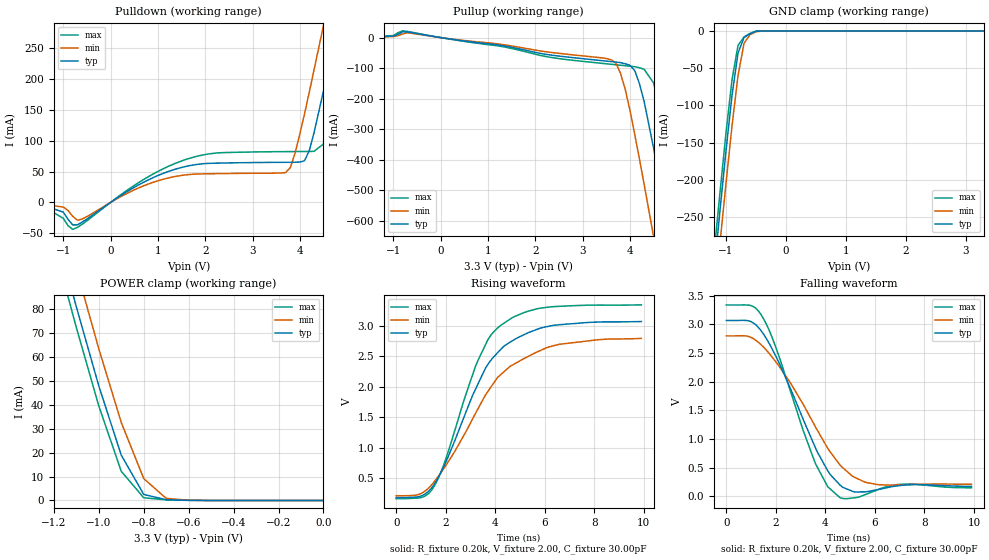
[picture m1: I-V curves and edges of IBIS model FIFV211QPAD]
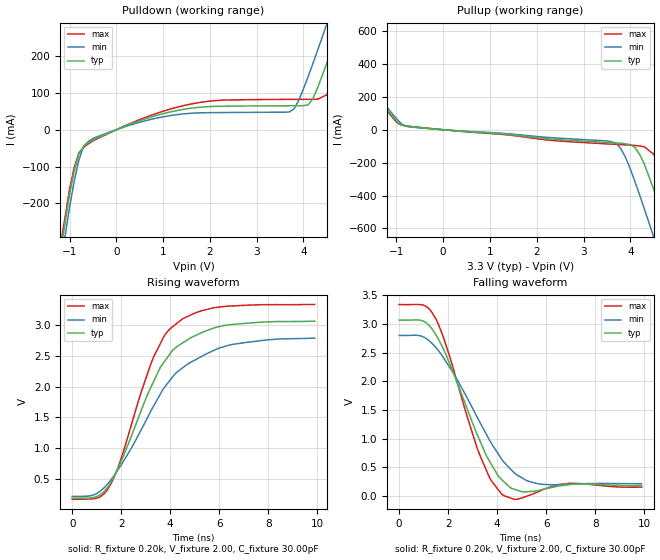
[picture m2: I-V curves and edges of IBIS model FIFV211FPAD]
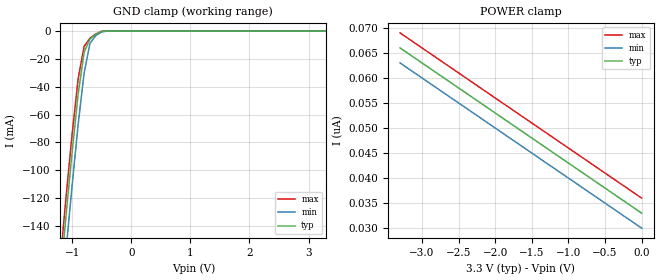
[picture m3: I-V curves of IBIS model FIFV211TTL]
| IBIS file i72v801.ibs created by s2ibis2 version 1.1
| North Carolina State University Electronics Research Laboratory  1995
[IBIS ver]   2.1
[File name]   i72v801.ibs
[File Rev]   1.0
[Date]   06/08/98
[Source]   Integrated Device Technology, Inc.
[Notes]   1. Temperatures: typ=25C, min=70C, max=0C 2. Cemos8_3.3v
   process. 3. Ramp rates based on 50 ohm load.
[Copyright]   Copyright 1998, Integrated Device Technology, Inc.
|   Component idt72V801
[Component]   idt72V801
[Manufacturer]   Integrated Device Technology
[Package]
| variable   typ   min   max
R_pkg   0.75   0.60   0.90
L_pkg   8.10nH   8.30nH   9.90nH
C_pkg   0.53pF   0.46pF   0.60pF
[Pin]  signal_name   model_name   R_pin   L_pin   C_pin
1   QA1   FIFV211QPAD
2   QA2   FIFV211QPAD
3   QA3   FIFV211QPAD
4   QA4   FIFV211QPAD
5   QA5   FIFV211QPAD
6   QA6   FIFV211QPAD
7   QA7   FIFV211QPAD
8   QA8   FIFV211QPAD
9   VCC   POWER
10   WENA2   FIFV211TTL
11   WCLKA   FIFV211TTL
12   WENAL1   FIFV211TTL
13   RSAL   FIFV211TTL
14   DA8   FIFV211TTL
15   DA7   FIFV211TTL
16   DA6   FIFV211TTL
17   DA5   FIFV211TTL
18   DA4   FIFV211TTL
19   DA3   FIFV211TTL
20   DA2   FIFV211TTL
21   DA1   FIFV211TTL
22   DA0   FIFV211TTL
23   PAFAL   FIFV211FPAD
24   PAEAL   FIFV211FPAD
25   WENB2   FIFV211TTL
26   WCLKB   FIFV211TTL
27   WENBL1   FIFV211TTL
28   RSBL   FIFV211TTL
29   DB8   FIFV211TTL
30   DB7   FIFV211TTL
31   DB6   FIFV211TTL
32   DB5   FIFV211TTL
33   DB4   FIFV211TTL
34   DB3   FIFV211TTL
35   DB2   FIFV211TTL
36   DB1   FIFV211TTL
37   DB0   FIFV211TTL
38   PAFBL   FIFV211FPAD
39   PAEBL   FIFV211FPAD
40   VCC   POWER
41   GND   GND
42   RENBL1   FIFV211TTL
43   RCLKB   FIFV211TTL
44   RENBL2   FIFV211TTL
45   OEBL   FIFV211TTL
46   EFBL   FIFV211FPAD
47   FFBL   FIFV211FPAD
48   QB0   FIFV211QPAD
49   QB1   FIFV211QPAD
50   QB2   FIFV211QPAD
51   QB3   FIFV211QPAD
52   QB4   FIFV211QPAD
53   QB5   FIFV211QPAD
54   QB6   FIFV211QPAD
55   QB7   FIFV211QPAD
56   QB8   FIFV211QPAD
57   GND   GND
58   RENAL1   FIFV211TTL
59   RCLKA   FIFV211TTL
60   RENAL2   FIFV211TTL
61   OEAL   FIFV211TTL
62   EFAL   FIFV211FPAD
63   FFAL   FIFV211FPAD
64   QA0   FIFV211QPAD
| Models and submodels in the file (3): FIFV211QPAD (3-state), FIFV211FPAD (Output), FIFV211TTL (Input)
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| FIN  FIN   dummy_model
| QIN  QIN   dummy_model
| QOEL QOEL   dummy_model
|   Model FIFV211QPAD
[Model]   FIFV211QPAD
Model_type   3-state
Polarity   Non-Inverting
Enable   Active-Low
Vmeas =  1.500V
C_comp   3.00pF   NA   NA
[Temperature Range]   25.00   70.00   0.000
[Voltage Range]   3.30V   3.00V   3.60V
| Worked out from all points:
|   slope of the pulldown table from 0 to 0.495 V, typ, clamps not added: 20.4 ohm
|   slope of the pullup table from 0 to 0.495 V, typ, clamps not added: 44.7 ohm
|   GND clamp passes 1 mA (typ) near -0.52 V on its own axis
|   POWER clamp passes 1 mA (typ) near -0.73 V on its own axis
|   rising waveform, R_fixture 0.20k, V_fixture 2.00, C_fixture 30.00pF: 20-80 % time 1.95ns typ, 2.41ns min, 1.64ns max; typ from 0.181 V to 3.07 V
|   falling waveform, R_fixture 0.20k, V_fixture 2.00, C_fixture 30.00pF: 20-80 % time 1.76ns typ, 2.17ns min, 1.5ns max; typ from 3.07 V to 0.177 V
[Pulldown]
| voltage   I(typ)   I(min)   I(max)
-3.3V     -1mA       -1mA       0A
-1.5V     -2.7mA     -2.1mA     -3.3mA
-800mV    -36.55mA   -22.69mA   -43.77mA
1.5V      56.64mA    43.75mA    67.16mA
3.7V      65mA       48.37mA    82.35mA
3.9V      65.11mA    80.12mA    82.43mA
4.1V      67.6mA     144mA      82.48mA
4.5V      181mA      287mA      94.75mA
4.7V      253mA      361mA      155mA
4.9V      326mA      435mA      225mA
5.1V      400mA      510mA      298mA
6.6V      966mA      1.076A     862mA
[Pullup]
| voltage   I(typ)   I(min)   I(max)
-3.3V     300uA      300uA      300uA
-800mV    19.13mA    12.44mA    22.38mA
3.6V      -78.68mA   -72.88mA   -87.52mA
3.7V      -80.24mA   -82.94mA   -89.09mA
3.9V      -85.87mA   -170mA     -92.22mA
4.1V      -108mA     -317mA     -95.4mA
4.3V      -210mA     -482mA     -104mA
4.5V      -363mA     -653mA     -149mA
4.7V      -531mA     -826mA     -270mA
4.9V      -703mA     -1A        -430mA
5.1V      -878mA     -1.176A    -601mA
6.6V      -2.207A    -2.508A    -1.926A
[GND_clamp]
| voltage   I(typ)   I(min)   I(max)
-3.3V     -2.171A    -2.212A    -2.149A
-1.2V     -323mA     -367mA     -298mA
-1.1V     -240mA     -284mA     -216mA
-1V       -160mA     -204mA     -136mA
-900mV    -86.07mA   -127mA     -65.05mA
-800mV    -29.34mA   -59.59mA   -19.24mA
-700mV    -8.788mA   -16.49mA   -7.804mA
-600mV    -3.672mA   -4.887mA   -3.17mA
-500mV    -365uA     -944uA     -138uA
-400mV    -14.29nA   -611nA     -4.611nA
3.3V      33nA       33.88nA    33nA
[POWER_clamp]
| voltage   I(typ)   I(min)   I(max)
-3.3V     901mA      915mA      893mA
-1.2V     116mA      132mA      107mA
-1.1V     80.92mA    96.84mA    72.29mA
-1V       47.89mA    63.39mA    39.51mA
-900mV    18.95mA    32.6mA     12.21mA
-800mV    2.533mA    9.147mA    1.14mA
-700mV    314uA      878uA      268uA
-600mV    64.82uA    96.03uA    58.5uA
0V        33nA       30nA       36nA
[Ramp]
| variable   typ   min   max
dV/dt_r   1.03/1.09n   0.87/1.27n   1.19/0.99n
dV/dt_f   1.35/1.45n   1.13/1.85n   1.54/1.17n
R_load = 50.00
[Rising Waveform]
R_fixture = 0.20k
V_fixture = 2.00
C_fixture = 30.00pF
R_dut = 0.75
L_dut = 8.10nH
C_dut = 0.53pF
| time   V(typ)   V(min)   V(max)
0s        181mV      211mV      165mV
1ns       207mV      250mV      183mV
1.5ns     380mV      424mV      346mV
2ns       761mV      708mV      812mV
3.2ns     1.956V     1.561V     2.333V
3.7ns     2.364V     1.92V      2.767V
4.2ns     2.601V     2.19V      2.998V
5.2ns     2.859V     2.468V     3.22V
6.4ns     3.007V     2.675V     3.312V
9.9ns     3.067V     2.791V     3.339V
[Falling Waveform]
R_fixture = 0.20k
V_fixture = 2.00
C_fixture = 30.00pF
R_dut = 0.75
L_dut = 8.10nH
C_dut = 0.53pF
| time   V(typ)   V(min)   V(max)
0s        3.068V     2.8V       3.338V
1ns       3.048V     2.773V     3.327V
1.5ns     2.831V     2.606V     3.1V
2ns       2.445V     2.345V     2.598V
3.6ns     846mV      1.212V     571mV
4.1ns     445mV      835mV      168mV
4.6ns     195mV      542mV      -23.03mV
6.1ns     119mV      207mV      115mV
7.3ns     201mV      207mV      218mV
9.9ns     177mV      213mV      152mV
|   Model FIFV211FPAD
[Model]   FIFV211FPAD
Model_type   Output
Vmeas =  1.500V
C_comp   3.00pF   NA   NA
[Temperature Range]   25.00   70.00   0.000
[Voltage Range]   3.30V   3.00V   3.60V
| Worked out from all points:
|   slope of the pulldown table from 0 to 0.495 V, typ, clamps not added: 20.4 ohm
|   slope of the pullup table from 0 to 0.495 V, typ, clamps not added: 44.7 ohm
|   rising waveform, R_fixture 0.20k, V_fixture 2.00, C_fixture 30.00pF: 20-80 % time 1.94ns typ, 2.4ns min, 1.63ns max; typ from 0.181 V to 3.07 V
|   falling waveform, R_fixture 0.20k, V_fixture 2.00, C_fixture 30.00pF: 20-80 % time 1.62ns typ, 2.05ns min, 1.36ns max; typ from 3.07 V to 0.176 V
[Pulldown]
| voltage   I(typ)   I(min)   I(max)
-3.3V     -2.793A    -2.213A    -2.149A
-1.5V     -582mA     -626mA     -558mA
-1V       -176mA     -211mA     -162mA
-800mV    -65.89mA   -82.28mA   -63.01mA
-400mV    -21.63mA   -18.48mA   -23.86mA
1.6V      58.46mA    44.74mA    69.8mA
3.7V      65mA       48.37mA    82.35mA
4.1V      67.6mA     144mA      82.48mA
4.5V      181mA      287mA      94.75mA
4.7V      253mA      361mA      155mA
5.1V      400mA      510mA      298mA
6.6V      966mA      1.076A     862mA
[Pullup]
| voltage   I(typ)   I(min)   I(max)
-3.3V     901mA      915mA      893mA
-2.5V     598mA      613mA      590mA
-900mV    29.8mA     38.77mA    28.31mA
3.6V      -78.68mA   -72.88mA   -87.52mA
3.9V      -85.87mA   -170mA     -92.22mA
4.1V      -108mA     -317mA     -95.4mA
4.3V      -210mA     -482mA     -104mA
4.5V      -363mA     -653mA     -149mA
4.7V      -531mA     -826mA     -270mA
4.9V      -703mA     -1A        -430mA
5.1V      -878mA     -1.176A    -601mA
6.6V      -2.207A    -2.508A    -1.926A
[Ramp]
| variable   typ   min   max
dV/dt_r   1.03/1.07n   0.87/1.29n   1.19/0.96n
dV/dt_f   1.35/1.23n   1.13/1.60n   1.54/1.03n
R_load = 50.00
[Rising Waveform]
R_fixture = 0.20k
V_fixture = 2.00
C_fixture = 30.00pF
R_dut = 0.75
L_dut = 8.10nH
C_dut = 0.53pF
| time   V(typ)   V(min)   V(max)
0s        181mV      211mV      165mV
1ns       210mV      260mV      183mV
1.5ns     393mV      443mV      363mV
2ns       788mV      728mV      837mV
3.3ns     2.067V     1.67V      2.468V
3.8ns     2.43V      2.009V     2.856V
4.1ns     2.595V     2.161V     2.978V
5.1ns     2.846V     2.454V     3.213V
6.4ns     3.009V     2.676V     3.312V
9.9ns     3.067V     2.791V     3.339V
[Falling Waveform]
R_fixture = 0.20k
V_fixture = 2.00
C_fixture = 30.00pF
R_dut = 0.75
L_dut = 8.10nH
C_dut = 0.53pF
| time   V(typ)   V(min)   V(max)
0s        3.068V     2.8V       3.338V
1ns       3.047V     2.771V     3.327V
1.5ns     2.812V     2.59V      3.088V
3.2ns     1.059V     1.362V     814mV
3.7ns     598mV      964mV      309mV
4.2ns     280mV      631mV      25.41mV
5ns       74.15mV    319mV      -37.61mV
5.7ns     96.8mV     209mV      77.59mV
7ns       200mV      204mV      221mV
9.9ns     176mV      212mV      154mV
|   Model FIFV211TTL
[Model]   FIFV211TTL
Model_type   Input
Vinl =  0.000V
Vinh =  3.000V
Vmeas =  1.500V
C_comp   3.00pF   NA   NA
[Temperature Range]   25.00   70.00   0.000
[Voltage Range]   3.30V   3.00V   3.60V
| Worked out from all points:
|   GND clamp passes 1 mA (typ) near -0.54 V on its own axis
[GND_clamp]
| voltage   I(typ)   I(min)   I(max)
-3.3V     -1.215A    -1.238A    -1.203A
-1.2V     -177mA     -201mA     -164mA
-1.1V     -130mA     -155mA     -117mA
-1V       -85.9mA    -110mA     -73.09mA
-900mV    -45.15mA   -67.03mA   -34.14mA
-800mV    -15.42mA   -30.38mA   -11.05mA
-700mV    -5.554mA   -8.773mA   -5.066mA
-600mV    -2.384mA   -3.102mA   -2.034mA
-500mV    -209uA     -595uA     -61.81uA
-400mV    -8.386nA   -263nA     -4.26nA
3.3V      33nA       33nA       33nA
[POWER_clamp]
| voltage   I(typ)   I(min)   I(max)
-3.3V     66nA       63nA       69nA
-3.2V     65nA       62nA       68nA
-3V       63nA       60nA       66nA
0V        33nA       30nA       36nA
